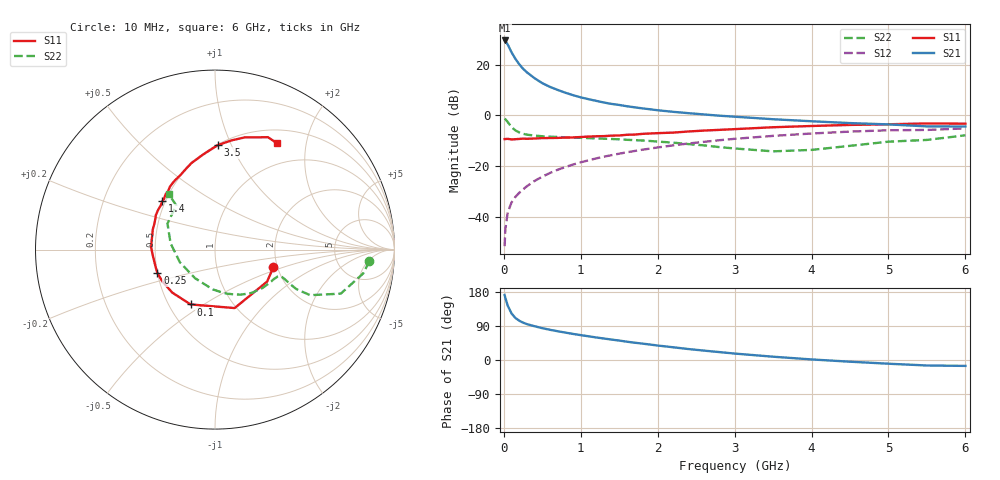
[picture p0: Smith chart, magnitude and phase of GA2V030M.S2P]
! Infineon Technologies  Discrete & RF Semiconductors
! BF775
! Si NPN RF Bipolar Junction Transistor in SOT23
! VCE = 2 V  IC = 30 mA
! Common Emitter S-Parameters:  May  1996
# GHz  S  MA  R  50
!  f  S11  S21  S12  S22
! GHz  MAG  ANG  MAG  ANG  MAG  ANG  MAG  ANG
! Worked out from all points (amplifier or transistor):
!   36 points, 10 MHz to 6 GHz, reference 50 ohm
!   highest |S21| = 29.6 dB at 10 MHz (marker M1)
!   |S21| within 3 dB of that: start of sweep to 72.98 MHz
!   unconditionally stable (mu >= 1): start of sweep to 15.19 MHz; 139.4 MHz to end of sweep
!   at 250 MHz: K = 1.25, MAG = 20.8 dB, |S12| = -29.3 dB
!   at 1.4 GHz: K = 1.36, MAG = 6.6 dB, |S12| = -15.7 dB
!   at 6 GHz: K = 1.09, MAG = -1.4 dB, |S12| = -5.1 dB
!   S11 on the Smith chart (normalised r, x): 10 MHz: 1.91, -0.42; 100 MHz: 0.64, -0.44; 250 MHz: 0.50, -0.15; 1.4 GHz: 0.48, +0.31; 3.5 GHz: 0.51, +0.89; 6 GHz: 0.67, +1.51
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0.01  0.3399 -16.6  30.25 171.6  0.0026 80.3  0.8623 -4.3
0.02  0.3407 -31.5  29.45 163.6  0.0057 82.6  0.8369 -9.1
0.05  0.3437 -71.4  25.19 143.7  0.012 68.6  0.7425 -19.3
0.1  0.3344 -114.0  17.69 122.8  0.019 64.1  0.5877 -25.6
0.15  0.3379 -134.9  13.15 111.0  0.0245 63.3  0.5043 -25.9
0.2  0.3425 -148.7  10.26 103.7  0.0295 66.0  0.4596 -24.6
0.25  0.3467 -157.7  8.326 98.6  0.0344 67.5  0.4318 -23.4
0.3  0.3446 -164.6  7.09 94.7  0.0398 69.3  0.4162 -22.7
0.4  0.3488 -175.4  5.417 89.1  0.0507 71.1  0.3983 -22.1
0.5  0.3557 178.2  4.33 84.0  0.0615 71.9  0.3863 -22.4
0.6  0.3568 171.4  3.653 79.7  0.0727 71.8  0.3796 -23.3
0.8  0.3644 162.2  2.803 72.3  0.0954 71.0  0.3684 -26.1
0.9  0.3666 157.5  2.505 68.8  0.1067 70.6  0.3636 -27.8
1.1  0.3816 149.6  2.09 62.6  0.1294 69.2  0.3551 -32.0
1.4  0.3976 137.5  1.686 53.9  0.1636 66.1  0.3413 -38.4
1.7  0.4172 128.8  1.443 45.6  0.1977 62.8  0.3234 -45.6
2.2  0.4564 115.3  1.176 33.6  0.2552 56.4  0.2893 -60.2
2.8  0.517 100.7  0.986 20.9  0.3225 48.1  0.2363 -83.5
3.5  0.5828 88.4  0.839 8.7  0.3933 37.5  0.1945 -125.0
4.5  0.6477 75.0  0.704 -4.5  0.4779 22.2  0.2501 171.9
5.5  0.6923 64.8  0.606 -14.5  0.5153 6.8  0.3273 131.2
6  0.6861 60.0  0.602 -15.6  0.5535 2.5  0.4038 129.8
